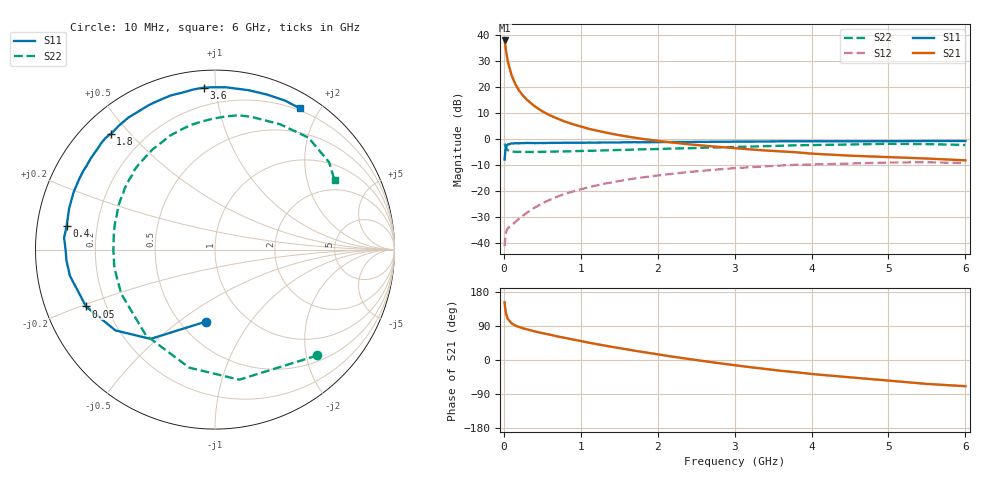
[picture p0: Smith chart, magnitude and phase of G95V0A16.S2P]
! SIEMENS Small Signal Semiconductors
! BFG235
! Si NPN RF Bipolar Junction Transistor in SOT223
! VCE = 5 V  IC = 160 mA
! Common Emitter S-Parameters:  July  1994
# GHz  S  MA  R  50
!  f  S11  S21  S12  S22
! GHz  MAG  ANG  MAG  ANG  MAG  ANG  MAG  ANG
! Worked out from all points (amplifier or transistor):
!   40 points, 10 MHz to 6 GHz, reference 50 ohm
!   highest |S21| = 37.9 dB at 10 MHz (marker M1)
!   |S21| within 3 dB of that: start of sweep to 24.17 MHz
!   unconditionally stable (mu >= 1): 436.8 MHz to 1.513 GHz
!   at 200 MHz: K = 0.82, MSG = 24.5 dB, |S12| = -30.5 dB
!   at 1.5 GHz: K = 1.00, MAG = 8.5 dB, |S12| = -16.1 dB
!   at 6 GHz: K = 0.89, MSG = 0.5 dB, |S12| = -9.2 dB
!   S11 on the Smith chart (normalised r, x): 10 MHz: 0.66, -0.63; 50 MHz: 0.13, -0.21; 400 MHz: 0.09, +0.08; 1.8 GHz: 0.08, +0.44; 3.6 GHz: 0.09, +0.93; 6 GHz: 0.17, +1.75
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0.01  0.4042 -97.2  78.14 152.2  0.0088 62.5  0.82 -46.0
0.02  0.6133 -125.8  61.26 133.2  0.014 48.1  0.7373 -79.4
0.03  0.7143 -140.9  47.98 121.4  0.0168 40.9  0.6733 -102.3
0.05  0.7853 -156.2  31.87 108.9  0.0193 34.0  0.6133 -128.9
0.1  0.8216 -169.8  16.82 96.9  0.0221 37.0  0.5776 -154.7
0.15  0.8301 -175.9  11.29 90.9  0.0256 44.5  0.5684 -165.4
0.2  0.8314 -179.2  8.45 87.0  0.0299 48.8  0.5684 -171.4
0.25  0.8369 177.9  6.807 83.6  0.034 51.6  0.5654 -175.6
0.3  0.8434 175.5  5.685 80.9  0.0386 54.8  0.5663 -179.2
0.4  0.8371 171.1  4.275 75.6  0.0482 57.3  0.5661 175.8
0.5  0.8392 167.5  3.415 70.9  0.0583 58.6  0.5702 171.6
0.7  0.8462 160.9  2.461 62.1  0.079 57.9  0.5775 164.2
0.9  0.8504 155.3  1.928 54.0  0.0988 55.1  0.5848 158.1
1.1  0.8549 149.2  1.582 45.8  0.1187 51.6  0.5958 151.9
1.4  0.8599 141.8  1.266 34.8  0.1471 45.7  0.6122 143.5
1.8  0.8678 132.0  1.008 21.3  0.1833 37.0  0.6362 132.6
2.2  0.8798 123.2  0.855 8.6  0.2166 28.1  0.6579 121.9
3.2  0.8931 102.0  0.635 -18.9  0.2884 4.9  0.717 96.1
3.6  0.9049 93.9  0.58 -28.5  0.3106 -5.0  0.7451 85.1
4.5  0.9076 78.1  0.48 -45.7  0.3394 -24.7  0.787 62.5
5.5  0.917 64.9  0.423 -63.1  0.358 -46.5  0.8007 37.5
6  0.9184 59.1  0.391 -69.2  0.3485 -54.8  0.7704 30.2
